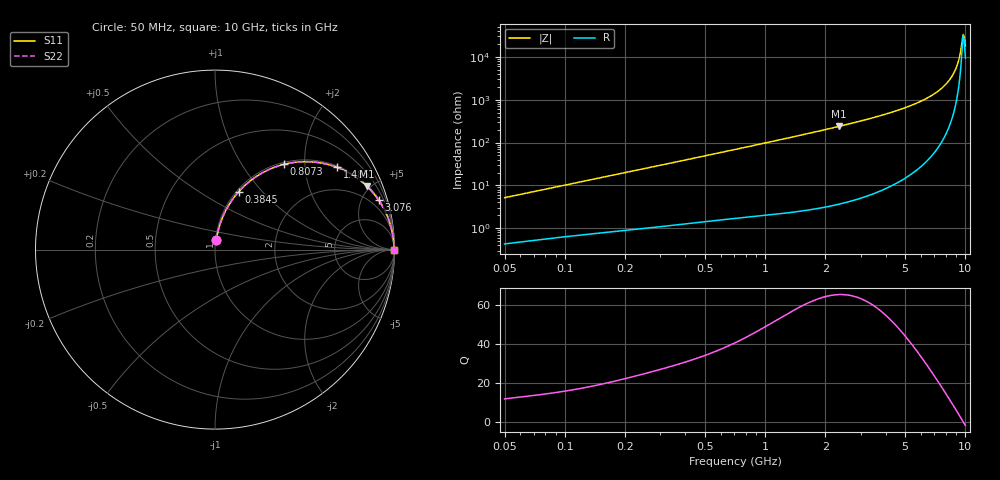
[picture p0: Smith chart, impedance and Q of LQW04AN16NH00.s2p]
!Murata Part Number: LQW04AN16NH00
!These Parameters are Measured in Series Mode Connection
!  o--[Z]--o
!Port1  Port2
!  o-------o
!Freq. Start=50[MHz] Stop=10[GHz], 401[Steps]
# Hz S RI R 50
!Freq.(Hz)	S 11(Real)	S 11(Imag)	S 21(Real)	S 21(Imag)	S 12(Real)	S 12(Imag)	S 22(Real)	S 22(Imag)
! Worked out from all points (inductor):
!   401 points, 50 MHz to 10 GHz, reference 50 ohm
!   read as one part in series: L = 16.3 nH near 51.34 MHz
!   highest Q = 65.4 at 2.329 GHz (marker M1), where L = 16.2 nH
!   self-resonance near 9.739 GHz
!   S11 on the Smith chart (normalised r, x): 50 MHz: 1.01, +0.10; 384.5 MHz: 1.02, +0.75; 807.3 MHz: 1.04, +1.57; 1.485 GHz: 1.05, +2.93; 3.076 GHz: 1.10, +6.57; 10 GHz: open
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5e7  0.00691 0.051  0.9931 -0.051  0.9931 -0.051  0.00691 0.051
1.214486e8  0.0213 0.1184  0.9787 -0.1184  0.9787 -0.1184  0.0213 0.1184
2.949953e8  0.0861 0.2625  0.9139 -0.2625  0.9139 -0.2625  0.0861 0.2625
3.844736e8  0.1325 0.3229  0.8675 -0.3229  0.8675 -0.3229  0.1325 0.3229
7.071068e8  0.3263 0.4568  0.6737 -0.4568  0.6737 -0.4568  0.3263 0.4568
8.07255e8  0.3853 0.4753  0.6147 -0.4753  0.6147 -0.4753  0.3853 0.4753
1.094763e9  0.5336 0.4892  0.4664 -0.4892  0.4664 -0.4892  0.5336 0.4892
1.484667e9  0.6794 0.4583  0.3206 -0.4583  0.3206 -0.4583  0.6794 0.4583
1.717543e9  0.7413 0.43  0.2587 -0.43  0.2587 -0.43  0.7413 0.43
2.329253e9  0.8459 0.3535  0.1541 -0.3535  0.1541 -0.3535  0.8459 0.3535
3.076244e9  0.9115 0.2761  0.0885 -0.2761  0.0885 -0.2761  0.9115 0.2761
4.171863e9  0.9567 0.1943  0.0433 -0.1943  0.0433 -0.1943  0.9567 0.1943
6.125686e9  0.9864 0.1014  0.0136 -0.1014  0.0136 -0.1014  0.9864 0.1014
6.993273e9  0.9917 0.0719  0.00826 -0.0719  0.00826 -0.0719  0.9917 0.0719
7.775012e9  0.9946 0.0488  0.00537 -0.0488  0.00537 -0.0488  0.9946 0.0488
8.307378e9  0.9959 0.0346  0.00413 -0.0346  0.00413 -0.0346  0.9959 0.0346
8.759398e9  0.9966 0.0234  0.00344 -0.0234  0.00344 -0.0234  0.9966 0.0234
8.994549e9  0.9968 0.0177  0.0032 -0.0177  0.0032 -0.0177  0.9968 0.0177
9.236013e9  0.997 0.0121  0.00301 -0.0121  0.00301 -0.0121  0.997 0.0121
9.610418e9  0.9971 0.00373  0.00286 -0.00373  0.00286 -0.00373  0.9971 0.00373
9.868415e9  0.9972 -0.00187  0.00284 0.00187  0.00284 0.00187  0.9972 -0.00187
1e10  0.9971 -0.00467  0.00285 0.00467  0.00285 0.00467  0.9971 -0.00467
